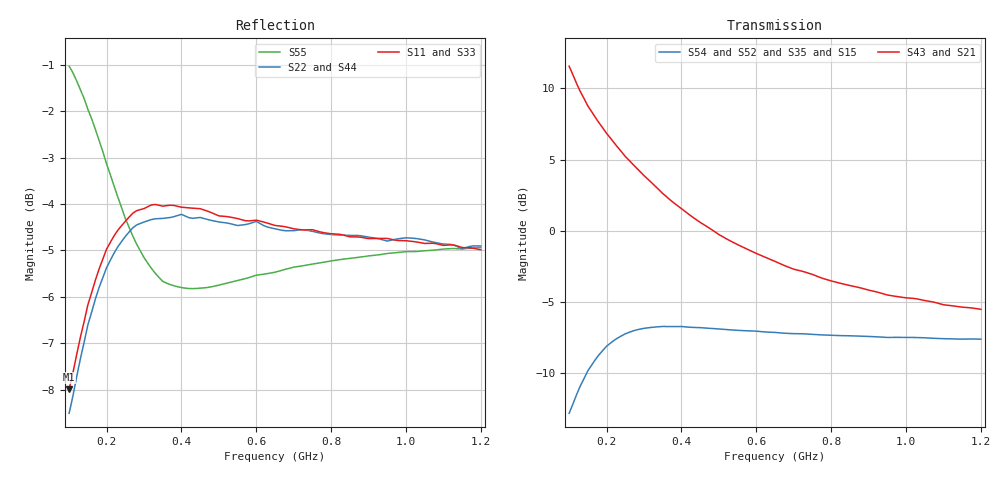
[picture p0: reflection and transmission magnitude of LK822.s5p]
!  POLYFET RF DEVICES
!  LK822  (EACH SIDE)
!  S PARAMETERS
!  VDS=12.5V, IDQ=400mA
!AWR Design Environment (2053) Wed Feb 04 14:59:38 2004
!freq-unit  param-type  data-format  keyword  impedance-ohms
# MHz  S  MA  R  50
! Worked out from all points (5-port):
!   111 points, 100 MHz to 1.2 GHz, reference 50 ohm
!   strongest paths, dB at 100 MHz, 370 MHz, 650 MHz, 930 MHz, 1.2 GHz:
!     S43: 11.6, 2.2, -2.2, -4.4, -5.5
!     S21: 11.6, 2.2, -2.2, -4.4, -5.5
!     S54: -12.8, -6.7, -7.2, -7.5, -7.6
!     S52: -12.8, -6.7, -7.2, -7.5, -7.6
!     S35: -12.5, -6.6, -7.2, -7.5, -7.7
!     S15: -12.5, -6.6, -7.2, -7.5, -7.7
!   lowest |S11| = -8.0 dB at 100 MHz (marker M1), VSWR 2.33, Z = 35.3 - j33.5 ohm
!   |S11| at or under -10 dB: nowhere
